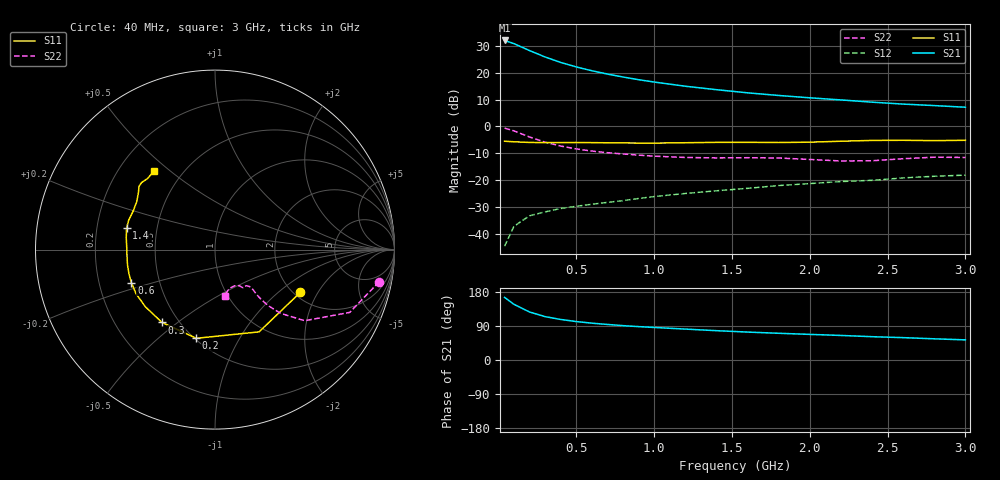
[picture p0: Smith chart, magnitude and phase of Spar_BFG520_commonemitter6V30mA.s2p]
! Filename:  BFG520L.S2P  Version:  2.1
! NXP part #: BFG520  Date: Feb 1992
! Bias condition: Vce=6V, Ic=30mA
! IN LINE PINNING: same data as with cross emitter pinning.
#  MHz  S  MA  R  50
! Freq  S11  S21  S12  S22  !GUM [dB]
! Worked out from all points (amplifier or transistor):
!   21 points, 40 MHz to 3 GHz, reference 50 ohm
!   highest |S21| = 31.9 dB at 40 MHz (marker M1)
!   |S21| within 3 dB of that: start of sweep to 170.8 MHz
!   unconditionally stable (mu >= 1): 795.1 MHz to end of sweep
!   at 300 MHz: K = 0.56, MSG = 28.8 dB, |S12| = -31.7 dB
!   at 1 GHz: K = 1.08, MAG = 19.5 dB, |S12| = -26.0 dB
!   at 3 GHz: K = 1.23, MAG = 9.7 dB, |S12| = -18.1 dB
!   S11 on the Smith chart (normalised r, x): 40 MHz: 2.16, -1.44; 200 MHz: 0.51, -0.68; 300 MHz: 0.41, -0.44; 600 MHz: 0.34, -0.17; 1.4 GHz: 0.33, +0.11; 3 GHz: 0.35, +0.44
40  0.532 -26.6  39.49 165.1  0.006 76.9  0.932 -11.1
100  0.52 -61.8  34.5 146.9  0.014 67.5  0.828 -25.0
200  0.505 -101.9  25.64 126.7  0.022 56.6  0.638 -38.4
300  0.502 -126.0  19.5 114.5  0.026 53.0  0.511 -44.1
400  0.502 -140.6  15.43 107.0  0.03 53.5  0.433 -46.4
500  0.504 -150.7  12.76 101.5  0.033 54.3  0.383 -47.2
600  0.501 -158.4  10.83 97.2  0.036 55.9  0.35 -47.2
700  0.498 -164.2  9.398 93.8  0.039 57.7  0.326 -46.9
800  0.495 -169.8  8.287 90.7  0.042 59.8  0.309 -46.5
900  0.492 -175.0  7.386 88.1  0.046 61.4  0.294 -46.5
1000  0.491 -179.7  6.68 85.9  0.05 62.7  0.281 -47.0
1200  0.499 172.3  5.587 81.6  0.057 64.3  0.266 -49.2
1400  0.507 166.4  4.82 77.4  0.064 65.5  0.261 -52.3
1600  0.508 161.2  4.21 73.7  0.071 67.8  0.263 -53.7
1800  0.504 155.0  3.763 70.5  0.08 67.7  0.26 -54.2
2000  0.511 148.6  3.403 67.6  0.087 68.8  0.244 -55.9
2200  0.532 143.3  3.11 64.8  0.095 68.7  0.229 -61.7
2400  0.551 140.2  2.826 61.5  0.1 69.8  0.231 -70.1
2600  0.554 137.6  2.602 59.0  0.111 69.6  0.252 -75.9
2800  0.546 133.5  2.442 55.9  0.119 68.1  0.269 -77.2
3000  0.554 128.0  2.274 53.1  0.125 68.9  0.266 -77.8
